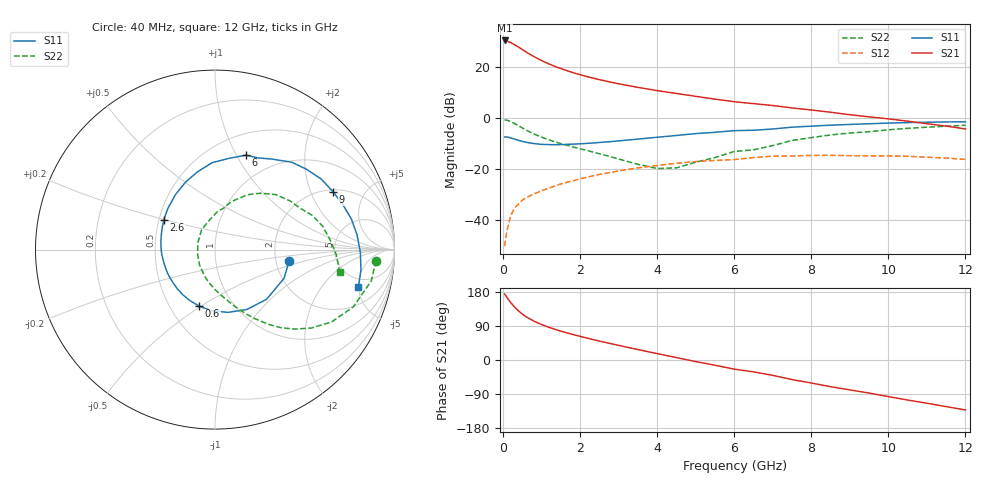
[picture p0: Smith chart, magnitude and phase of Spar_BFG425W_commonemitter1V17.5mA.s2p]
! Filename: 117bfg425.001
! BFG425W Field C1
! V1=8.701E-001V,V2=1.000E+000V, I1=2.655E-004A, I2=1.753E-002A
# GHz  S  MA  R 50
!  S11  S21  S12  S22
!Freq(GHz)  Mag  Ang  Mag  Ang  Mag  Ang  Mag  Ang
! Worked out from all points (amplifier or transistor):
!   44 points, 40 MHz to 12 GHz, reference 50 ohm
!   highest |S21| = 30.3 dB at 40 MHz (marker M1)
!   |S21| within 3 dB of that: start of sweep to 441.3 MHz
!   unconditionally stable (mu >= 1): 1.282 GHz to end of sweep
!   at 700 MHz: K = 0.75, MSG = 27.8 dB, |S12| = -30.8 dB
!   at 2.4 GHz: K = 1.16, MAG = 16.5 dB, |S12| = -22.6 dB
!   at 12 GHz: K = 1.36, MAG = 2.4 dB, |S12| = -16.4 dB
!   S11 on the Smith chart (normalised r, x): 40 MHz: 2.36, -0.38; 600 MHz: 0.70, -0.49; 2.6 GHz: 0.53, +0.19; 6 GHz: 0.72, +1.10; 9 GHz: 2.10, +2.92; 12 GHz: 3.77, -4.97
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0.04  0.417 -9.1  32.56 173.9  0.003 79.3  0.899 -4.0
0.1  0.417 -22.5  31.71 165.2  0.006 81.4  0.888 -11.4
0.2  0.399 -43.9  29.48 151.2  0.012 73.6  0.834 -22.5
0.3  0.378 -62.1  26.91 139.8  0.017 68.4  0.765 -31.8
0.4  0.357 -78.5  24.14 129.8  0.02 64.1  0.692 -39.2
0.5  0.341 -93.4  21.59 121.1  0.024 60.9  0.626 -45.0
0.6  0.327 -105.6  19.32 114.1  0.027 58.9  0.569 -49.9
0.7  0.317 -116.1  17.39 108.1  0.029 57.1  0.519 -53.8
0.8  0.309 -125.5  15.75 102.7  0.032 55.9  0.477 -57.1
0.9  0.303 -133.7  14.35 97.9  0.034 55.0  0.443 -60.1
1.2  0.295 -153.7  11.22 85.9  0.042 52.8  0.364 -67.6
1.6  0.297 -173.9  8.603 73.2  0.052 49.6  0.293 -76.1
2.2  0.312 163.1  6.307 57.3  0.068 43.5  0.224 -89.7
2.6  0.329 150.2  5.33 47.7  0.079 38.8  0.187 -100.4
3.5  0.378 125.5  3.911 27.6  0.103 26.4  0.121 -135.4
4.5  0.445 102.5  2.964 6.4  0.127 11.1  0.103 157.0
6  0.554 71.8  2.046 -24.1  0.15 -13.5  0.216 85.5
6.5  0.564 65.0  1.877 -31.3  0.164 -17.5  0.233 78.9
8.5  0.71 33.7  1.273 -70.4  0.182 -53.6  0.456 42.2
9  0.733 26.0  1.138 -78.9  0.179 -61.5  0.497 33.3
10.5  0.796 5.8  0.851 -105.7  0.174 -87.0  0.615 12.0
12  0.826 -14.7  0.598 -131.7  0.151 -114.9  0.706 -10.1
